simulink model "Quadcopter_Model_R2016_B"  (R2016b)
settings: Solver=VariableStepAuto  StartTime=0.0  StopTime=runtime  RelTol=1e-3
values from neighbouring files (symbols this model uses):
  delta_T = [ 0,  0,  9.404e-04 ]    [modelParameters.m]
  g = 9.81    [modelParameters.m]
  height_controlled_o = (((Rm*If        + (((omega0_o * 2 * Rm * Kv * Kq      * Kd + 1)^2) - 1)/(4* Rm*Kv^2*Kq      * Kd))/Vb)*(Pmax - Pmin) + Pmin)    [modelParameters.m]
  If = 0.3836    [modelParameters.m]
  Jreq = 4.2012e-05    [modelParameters.m]
  Jxx = 0.0110    (= 0.011)    [modelParameters.m]
  Jyy = 0.0116    [modelParameters.m]
  Jzz = 0.0223    [modelParameters.m]
  Kd = 1.4852e-07    [modelParameters.m]
  Kh = 3.4574e-04    (= 0.00034574)    [modelParameters.m]
  Kq = 96.3422    [modelParameters.m]
  Kt = 1.2007e-05    [modelParameters.m]
  Kv = 96.3422    [modelParameters.m]
  m = 1.216    [modelParameters.m]
  omega0_o = sqrt((m*g)/(4*Kt))    [modelParameters.m]
  omega1_o = sqrt((m*g)/(4*Kt))    [modelParameters.m]
  omega2_o = sqrt((m*g)/(4*Kt))    [modelParameters.m]
  omega3_o = sqrt((m*g)/(4*Kt))    [modelParameters.m]
  pitch_o = 0    [modelParameters.m]
  pitchrate_o = 0    [modelParameters.m]
  Pmax = 1    [modelParameters.m]
  Pmin = 0    [modelParameters.m]
  r_oc = [ 0 ; 0 ; 0 ]    [modelParameters.m]
  rhx = 0.16    [modelParameters.m]
  rhy = 0.16    [modelParameters.m]
  rhz = 0.03    [modelParameters.m]
  Rm = 0.235    [modelParameters.m]
  roll_o = 0    [modelParameters.m]
  rollrate_o = 0    [modelParameters.m]
  Tc = 0.01    [modelParameters.m]
  Tq = 0.005    [modelParameters.m]
  Vb = 12.3    [modelParameters.m]
  x_controlled_o = 0    [modelParameters.m]
  x_o = 0    [modelParameters.m]
  x_vel_o = 0    [modelParameters.m]
  y_controlled_o = 0    [modelParameters.m]
  y_o = 0    [modelParameters.m]
  y_vel_o = 0    [modelParameters.m]
  yaw_controlled_o = 0    [modelParameters.m]
  yaw_o = 0    [modelParameters.m]
  yawrate_o = 0    [modelParameters.m]
  z_o = 0    [modelParameters.m]
  z_vel_o = 0    [modelParameters.m]
undefined symbols (not defined in the file or in its folder): Ki, Kp, Ts
libraries: simulink x16, Derivative x13, dsparch4 x3, vrlib x1
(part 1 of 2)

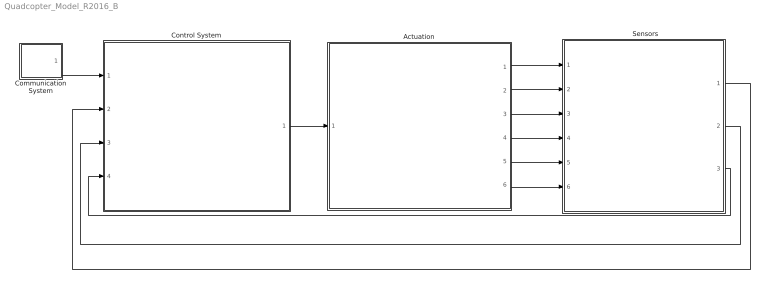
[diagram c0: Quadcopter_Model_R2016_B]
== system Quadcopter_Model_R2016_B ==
  "     Sensors   " : Subsystem
  Actuation : Subsystem
  Communication System : Subsystem
  Control System : Subsystem
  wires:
  Control System/1(P) -> Actuation/1(P)
  Actuation/6(B_g) -> "     Sensors   "/6(B_g)
  Actuation/5(B_vo_dot) -> "     Sensors   "/5(B_vo_dot)
  Actuation/4(E_ro) -> "     Sensors   "/4(E_ro)
  Actuation/3(B_vo) -> "     Sensors   "/3(B_vo)
  Actuation/1(B_omega) -> "     Sensors   "/1(B_Omega)
  "     Sensors   "/3(current_position) -> Control System/4(current_position)
  "     Sensors   "/2(euler_rates) -> Control System/3(euler_rates)
  "     Sensors   "/1(euler_angles_filtered) -> Control System/2(euler_angles_filtered)
  Actuation/2(euler_angles) -> "     Sensors   "/2(euler_angles)
  Communication System/1(setpoints) -> Control System/1(setpoints)

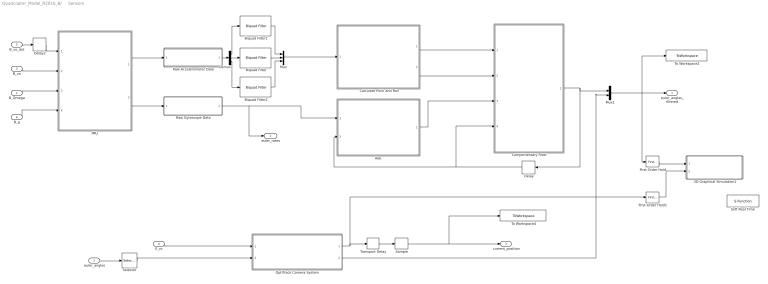
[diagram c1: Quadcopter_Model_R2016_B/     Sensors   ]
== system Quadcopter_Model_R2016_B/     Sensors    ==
  B_Omega : Inport
  euler_angles : Inport  Port=2
  B_vo : Inport  Port=3
  E_ro : Inport  Port=4
  B_vo_dot : Inport  Port=5
  B_g : Inport  Port=6
  3D Graphical Simulation1 : Subsystem
  "Aeb " : MATLAB Function  TreatAsAtomicUnit=on
  Biquad Filter : dsparch4/Biquad Filter  IIRFiltStruct=Direct form II  CoeffSource=Specify via dialog  BiQuadCoeffs=accel_SOS_Matrix  a0Flag=Warning  IC=0  ICnum=0  ICden=0  InputProcessing=Columns as channels (frame based)  denAccumFracLength=30  denProdOutputFracLength=30  secondMemoryFracLength=15  roundingMode=Floor  overflowMode=off  ScaleValues=1  optimizeScaleValues=on  ScaleValueMode=Specify via input port (g)  scaleValueFracLength=14  FilterSource=Specify via dialog  FilterObject=BQF
  Biquad Filter1 : dsparch4/Biquad Filter  IIRFiltStruct=Direct form II  CoeffSource=Specify via dialog  BiQuadCoeffs=accel_SOS_Matrix  a0Flag=Warning  IC=0  ICnum=0  ICden=0  InputProcessing=Columns as channels (frame based)  denAccumFracLength=30  denProdOutputFracLength=30  secondMemoryFracLength=15  roundingMode=Floor  overflowMode=off  ScaleValues=1  optimizeScaleValues=on  ScaleValueMode=Specify via input port (g)  scaleValueFracLength=14  FilterSource=Specify via dialog  FilterObject=BQF
  Biquad Filter2 : dsparch4/Biquad Filter  IIRFiltStruct=Direct form II  CoeffSource=Specify via dialog  BiQuadCoeffs=accel_SOS_Matrix  a0Flag=Warning  IC=0  ICnum=0  ICden=0  InputProcessing=Columns as channels (frame based)  denAccumFracLength=30  denProdOutputFracLength=30  secondMemoryFracLength=15  roundingMode=Floor  overflowMode=off  ScaleValues=1  optimizeScaleValues=on  ScaleValueMode=Specify via input port (g)  scaleValueFracLength=14  FilterSource=Specify via dialog  FilterObject=BQF
  Calculate Pitch and Roll : MATLAB Function  TreatAsAtomicUnit=on
  Complimentary Filter : MATLAB Function  TreatAsAtomicUnit=on
  Delay : Delay  DelayLength=1  InitialCondition=0
  Delay2 : Delay  DelayLength=1  InitialCondition=0  SampleTime=Tq
  Demux : Demux  Outputs=3
  First-Order Hold : simulink/Discrete/First-Order Hold  DisableCoverage=on  Ts=5e-3
  First-Order Hold1 : simulink/Discrete/First-Order Hold  DisableCoverage=on  Ts=5e-3
  "IMU " : Subsystem
  Mux : Mux  Inputs=3
  Mux1 : Mux  Inputs=2
  "OptiTrack Camera System " : Subsystem
  Raw Accelerometer Data : Subsystem  Variant=on
  Raw Gyroscope Data : Subsystem  Variant=on
  Sample : ZeroOrderHold  SampleTime=Tc
  Selector : Selector  InputPortWidth=3  IndexOptions=Index vector (dialog)  Indices=[3]  OutputSizes=1
  Soft Real Time : S-Function  Commented=on  FunctionName=sfun_time  Parameters=x  SFunctionDeploymentMode=off  EnableBusSupport=off
  To Workspace2 : ToWorkspace  VariableName=angle_IMU_reading  SaveFormat=Structure With Time  SampleTime=Tq
  To Workspace4 : ToWorkspace  VariableName=position_model  SaveFormat=Structure With Time  SampleTime=Tc
  Transport Delay : TransportDelay  DelayTime=6e-3
  euler_angles_filtered : Outport
  euler_rates : Outport  Port=2
  current_position : Outport  Port=3
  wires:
  "IMU "/1(accelerometer) -> Raw Accelerometer Data/1(raw_accel_model)
  "IMU "/2(gyroscope) -> Raw Gyroscope Data/1(raw_gyro_model)
  B_vo/1 -> "IMU "/2(B_vo)
  B_Omega/1 -> "IMU "/3(B_Omega)
  B_g/1 -> "IMU "/4(B_g)
  Calculate Pitch and Roll/2(accel_roll) -> Complimentary Filter/2(accel_roll)
  Calculate Pitch and Roll/1(accel_pitch) -> Complimentary Filter/1(accel_pitch)
  First-Order Hold/1 -> 3D Graphical Simulation1/1("Euler Angles ")
  E_ro/1 -> "OptiTrack Camera System "/1(E_ro)
  First-Order Hold1/1 -> 3D Graphical Simulation1/2(Displacement)
  B_vo_dot/1 -> Delay2/1
  Delay2/1 -> "IMU "/1(B_vo_dot)
  "OptiTrack Camera System "/1(E_ro_camera) -> Transport Delay/1, First-Order Hold1/1
  Transport Delay/1 -> Sample/1
  Sample/1 -> To Workspace4/1, current_position/1
  Raw Gyroscope Data/1(raw_gyro) -> "Aeb "/1(gyro_reading), euler_rates/1
  Delay/1 -> Complimentary Filter/4(prev_euler_angles), "Aeb "/2(euler_angles_filtered)
  "OptiTrack Camera System "/2(yaw_camera) -> Mux1/2
  "Aeb "/1(euler_rates_IMU) -> Complimentary Filter/3(euler_rates_gyro)
  Raw Accelerometer Data/1(raw_accel) -> Demux/1
  Demux/2 -> Biquad Filter/1
  Demux/1 -> Biquad Filter1/1
  Demux/3 -> Biquad Filter2/1
  Biquad Filter/1 -> Mux/2
  Biquad Filter1/1 -> Mux/1
  Biquad Filter2/1 -> Mux/3
  Mux/1 -> Calculate Pitch and Roll/1(accel_reading)
  Complimentary Filter/1(euler_angles_IMU) -> Mux1/1, Delay/1
  euler_angles/1 -> Selector/1
  Selector/1 -> "OptiTrack Camera System "/2(yaw)
  Mux1/1 -> To Workspace2/1, First-Order Hold/1, euler_angles_filtered/1

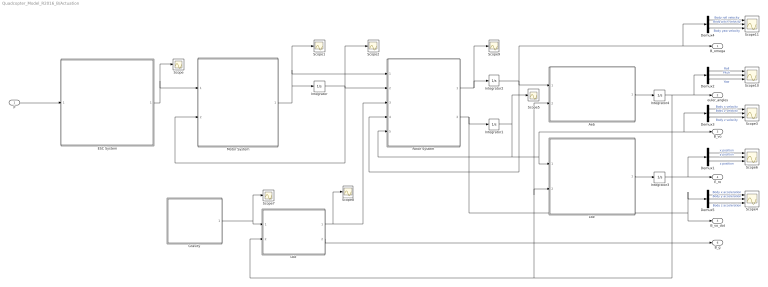
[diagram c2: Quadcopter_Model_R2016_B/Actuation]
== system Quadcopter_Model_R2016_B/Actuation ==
  P : Inport
  "Aeb " : MATLAB Function  TreatAsAtomicUnit=on
  Demux{1..5} (5 alike) : Demux  Outputs=3
  ESC System : MATLAB Function  TreatAsAtomicUnit=on
  "Gravity " : MATLAB Function  TreatAsAtomicUnit=on
  Integrator : Integrator  InitialCondition=[omega0_o, omega1_o, omega2_o, omega3_o]
  Integrator1 : Integrator  InitialCondition=[x_vel_o; y_vel_o; z_vel_o]
  Integrator2 : Integrator  InitialCondition=[rollrate_o; pitchrate_o; yawrate_o]
  Integrator3 : Integrator  InitialCondition=[x_o; y_o; z_o]
  Integrator4 : Integrator  InitialCondition=[roll_o; pitch_o; yaw_o]  ContinuousStateAttributes=['phi' 'theta' 'psi']
  "Lbe " : MATLAB Function  TreatAsAtomicUnit=on
  "Lbe " : MATLAB Function  TreatAsAtomicUnit=on
  Motor System : MATLAB Function  TreatAsAtomicUnit=on
  "Rotor System " : MATLAB Function  TreatAsAtomicUnit=on
  Scope{,1..2,5,7..9} (7 alike) : Scope
  Scope{3..4,6,10..11} (5 alike) : Scope  NumInputPorts=3
  B_omega : Outport
  euler_angles : Outport  Port=2
  B_vo : Outport  Port=3
  E_ro : Outport  Port=4
  B_vo_dot : Outport  Port=5
  B_g : Outport  Port=6
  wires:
  ESC System/1(Vb_eff) -> Scope/1, Motor System/1(Vb_eff)
  "Rotor System "/1(B_omega_dot) -> Scope9/1, Integrator2/1
  Integrator2/1 -> "Rotor System "/4(B_omega), B_omega/1, Demux4/1, "Aeb "/1(B_omega)
  "Aeb "/1(euler_rates) -> Integrator4/1
  "Lbe "/1(E_ro) -> Integrator3/1
  Integrator3/1 -> Demux1/1, E_ro/1
  "Lbe "/1(B_Fg) -> Scope8/1, "Rotor System "/3(B_Fg)
  "Lbe "/2(B_g) -> B_g/1
  Demux1/2 -> Scope6/2  "y position"
  Demux1/1 -> Scope6/1  "x position"
  Demux1/3 -> Scope6/3  "z position"
  Demux2/2 -> Scope10/2  "Pitch"
  Demux2/1 -> Scope10/1  "Roll"
  Demux2/3 -> Scope10/3  "Yaw"
  Demux4/2 -> Scope11/2  "Body pitch velocity"
  Demux4/1 -> Scope11/1  "Body roll velocity"
  Demux4/3 -> Scope11/3  "Body yaw velocity"
  Demux3/2 -> Scope3/2  "Body y velocity"
  Demux3/1 -> Scope3/1  "Body x velocity"
  Demux3/3 -> Scope3/3  "Body z velocity"
  Demux5/2 -> Scope4/2  "Body y acceleration"
  Demux5/1 -> Scope4/1  "Body x acceleration"
  Demux5/3 -> Scope4/3  "Body z acceleration"
  Integrator1/1 -> Scope5/1, "Rotor System "/5(B_vo), "Lbe "/1(B_vo), Demux3/1, B_vo/1
  "Rotor System "/2(B_vo_dot) -> Demux5/1, B_vo_dot/1, Integrator1/1
  Integrator4/1 -> euler_angles/1, Demux2/1, "Lbe "/2(euler_angles), "Aeb "/2(euler_angles), "Lbe "/2(euler_angles)
  P/1 -> ESC System/1(P)
  "Gravity "/1(E_Fg) -> Scope7/1, "Lbe "/1(E_Fg)
  Integrator/1 -> Motor System/2(w), "Rotor System "/2(w), Scope2/1
  Motor System/1(w_dot) -> Integrator/1, Scope1/1, "Rotor System "/1(w_dot)

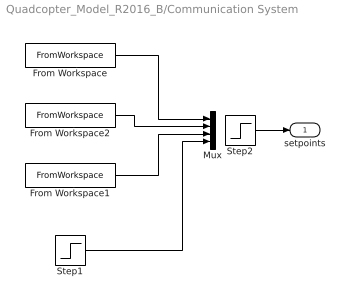
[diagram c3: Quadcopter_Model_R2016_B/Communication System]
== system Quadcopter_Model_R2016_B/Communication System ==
  From Workspace : FromWorkspace  Commented=on  VariableName=x_setpoint_model  SampleTime=Tq  Interpolate=off  OutputAfterFinalValue=Holding final value
  From Workspace1 : FromWorkspace  Commented=on  VariableName=z_setpoint_model  SampleTime=Tq  Interpolate=off  OutputAfterFinalValue=Holding final value
  From Workspace2 : FromWorkspace  Commented=on  VariableName=y_setpoint_model  SampleTime=Tq  Interpolate=off  OutputAfterFinalValue=Holding final value
  Mux : Mux
  Step1 : Step  After=0  SampleTime=0
  Step2 : Step  Before=[0,0,0,0]  After=[1,1,-1,0]  SampleTime=0
  setpoints : Outport
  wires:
  From Workspace/1 -> Mux/1
  From Workspace2/1 -> Mux/2
  From Workspace1/1 -> Mux/3
  Step1/1 -> Mux/4
  Step2/1 -> setpoints/1

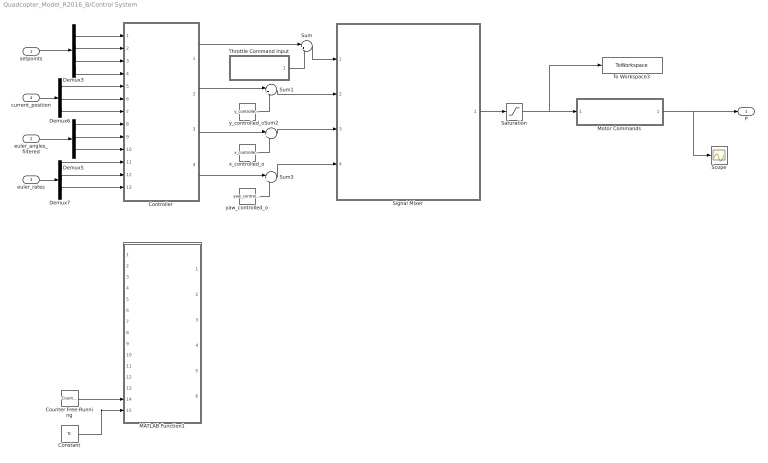
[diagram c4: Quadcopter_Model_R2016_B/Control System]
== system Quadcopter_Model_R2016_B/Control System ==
  setpoints : Inport
  euler_angles_filtered : Inport  Port=2
  euler_rates : Inport  Port=3
  current_position : Inport  Port=4
  Constant : Constant  Value=Tc  SampleTime=Tc
  Controller : Subsystem
  Counter Free-Running : simulink/Sources/Counter Free-Running  NumBits=32  tsamp=Tc
  Demux3 : Demux
  Demux5 : Demux  Outputs=3
  Demux6 : Demux  Outputs=3
  Demux7 : Demux  Outputs=3
  MATLAB Function1 : MATLAB Function  Commented=on  TreatAsAtomicUnit=on  SystemSampleTime=Tq
  Motor Commands : Subsystem  Variant=on
  Saturation : Saturate  UpperLimit=Pmax*ones(4,1)  LowerLimit=Pmin*ones(4,1)
  Scope : Scope
  Signal Mixer : MATLAB Function  TreatAsAtomicUnit=on
  Sum{,1..3} (4 alike) : Sum  Inputs=|++
  Throttle Command Input : Subsystem  Variant=on
  To Workspace3 : ToWorkspace  VariableName=motorCommands  SaveFormat=Structure With Time  SampleTime=Tq
  x_controlled_o : Constant  Value=x_controlled_o
  y_controlled_o : Constant  Value=y_controlled_o
  yaw_controlled_o : Constant  Value=yaw_controlled_o
  P : Outport
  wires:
  y_controlled_o/1 -> Sum1/2
  x_controlled_o/1 -> Sum2/2
  yaw_controlled_o/1 -> Sum3/2
  Signal Mixer/1(P) -> Saturation/1
  Counter Free-Running/1 -> MATLAB Function1/14(vrpn_id)
  Constant/1 -> MATLAB Function1/15(Tc)
  Sum1/1 -> Signal Mixer/2(y_controlled)
  Sum2/1 -> Signal Mixer/3(x_controlled)
  Sum3/1 -> Signal Mixer/4(yaw_controlled)
  Motor Commands/1(z_command) -> P/1, Scope/1
  Saturation/1 -> To Workspace3/1, Motor Commands/1(z_command_model)
  setpoints/1 -> Demux3/1
  current_position/1 -> Demux6/1
  euler_angles_filtered/1 -> Demux5/1
  euler_rates/1 -> Demux7/1
  Demux3/1 -> Controller/1(x_setpoint)
  Demux3/2 -> Controller/2(y_setpoint)
  Demux3/3 -> Controller/3(z_setpoint)
  Demux3/4 -> Controller/4(yaw_setpoint)
  Demux6/1 -> Controller/5(x_position)
  Demux6/2 -> Controller/6(y_position)
  Demux6/3 -> Controller/7(z_position)
  Demux5/1 -> Controller/8(roll)
  Demux5/2 -> Controller/9(pitch)
  Demux5/3 -> Controller/10(yaw)
  Demux7/1 -> Controller/11(roll_rate)
  Demux7/2 -> Controller/12(pitch_rate)
  Demux7/3 -> Controller/13(yaw_rate)
  Controller/1(height_controlled) -> Sum/1
  Controller/2(y_controlled) -> Sum1/1
  Controller/3(x_controlled) -> Sum2/1
  Controller/4(yaw_controlled) -> Sum3/1
  Throttle Command Input/1(z_command) -> Sum/2
  Sum/1 -> Signal Mixer/1(height_controlled)

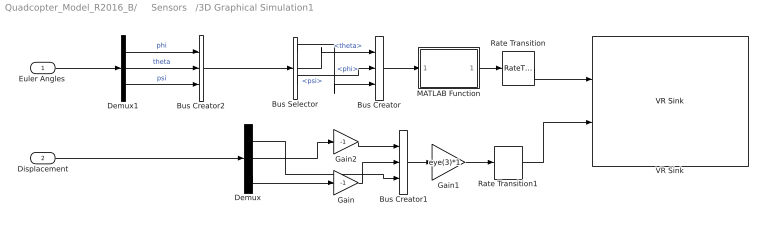
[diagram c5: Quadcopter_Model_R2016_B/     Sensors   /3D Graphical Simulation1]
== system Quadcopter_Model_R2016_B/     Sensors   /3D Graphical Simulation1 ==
  "Euler Angles " : Inport
  Displacement : Inport  Port=2
  Bus Creator : BusCreator  Inputs=3
  Bus Creator1 : BusCreator  Inputs=3
  Bus Creator2 : BusCreator  Inputs=3
  Bus Selector : BusSelector  OutputSignals=phi,theta,psi
  Demux : Demux  Outputs=3
  Demux1 : Demux  Outputs=3
  Gain : Gain  Gain=-1
  Gain1 : Gain  Gain=eye(3)*1  Multiplication=Matrix(K*u)
  Gain2 : Gain  Gain=-1
  MATLAB Function : MATLAB Function  TreatAsAtomicUnit=on
  Rate Transition : RateTransition  OutPortSampleTime=0.06
  Rate Transition1 : RateTransition  OutPortSampleTime=0.06
  VR Sink : vrlib/VR Sink  InstantiateOnLoad=on  SampleTime=-1  ViewEnable=on  RemoteChange=off  RemoteView=off  FieldsWritten=Helicopter.rotation.4.1.1.double#Helicopter.translation.3.1.1.double  WorldFileName=quadrotor_world_ucart.wrl  AutoView=on  VideoDimensions=[]  AllowVariableSize=off
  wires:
  Bus Creator2/1 -> Bus Selector/1
  Demux/1 -> Bus Creator1/3
  Gain/1 -> Bus Creator1/2
  Gain2/1 -> Bus Creator1/1
  Rate Transition1/1 -> VR Sink/2
  Rate Transition/1 -> VR Sink/1
  Demux/3 -> Gain/1
  Demux/2 -> Gain2/1
  Bus Creator1/1 -> Gain1/1
  Bus Selector/1 -> Bus Creator/3  "<phi>"
  Bus Selector/3 -> Bus Creator/2  "<psi>"
  Bus Selector/2 -> Bus Creator/1  "<theta>"
  Gain1/1 -> Rate Transition1/1
  Demux1/3 -> Bus Creator2/3  "psi"
  Demux1/2 -> Bus Creator2/2  "theta"
  Demux1/1 -> Bus Creator2/1  "phi"
  Bus Creator/1 -> MATLAB Function/1(u)
  MATLAB Function/1(y) -> Rate Transition/1
  Displacement/1 -> Demux/1
  "Euler Angles "/1 -> Demux1/1

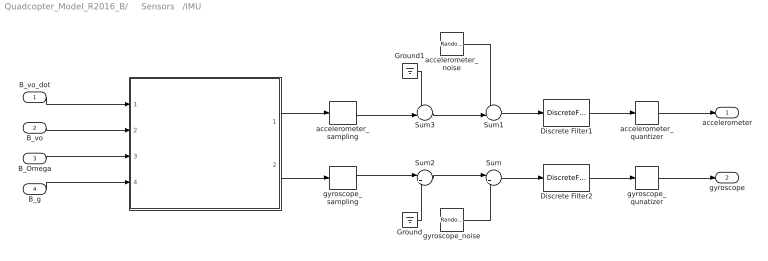
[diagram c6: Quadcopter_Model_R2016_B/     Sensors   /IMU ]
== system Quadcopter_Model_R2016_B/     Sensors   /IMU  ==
  B_vo_dot : Inport
  B_vo : Inport  Port=2
  B_Omega : Inport  Port=3
  B_g : Inport  Port=4
  " " : MATLAB Function  TreatAsAtomicUnit=on
  Discrete Filter1 : DiscreteFilter  Numerator=[0 0.749]  Denominator=[1 -0.251]  InitialStates=[0, 0, -1]  SampleTime=Tq
  Discrete Filter2 : DiscreteFilter  Numerator=[0 0.7327]  Denominator=[1 -0.2673]  SampleTime=Tq
  Ground : Ground
  Ground1 : Ground
  Sum : Sum  Inputs=|++
  Sum1 : Sum  Inputs=++|
  Sum2 : Sum  Inputs=|++
  Sum3 : Sum  Inputs=++|
  accelerometer_noise : RandomNumber  Mean=zeros(3,1)  Variance=[ 3e-7 ; 3.3e-7 ; 7.2e-7 ]  Seed=[0,1,2]  SampleTime=Tq
  accelerometer_quantizer : Quantizer  QuantizationInterval=2.4400e-04
  accelerometer_sampling : ZeroOrderHold  SampleTime=Tq
  gyroscope_noise : RandomNumber  Mean=zeros(3,1)  Variance=[ 2.2e-8 ; 1.1e-7 ; 2.4e-8 ]  Seed=[0,1,2]  SampleTime=Tq
  gyroscope_qunatizer : Quantizer  QuantizationInterval=1.1e-3
  gyroscope_sampling : ZeroOrderHold  SampleTime=Tq
  accelerometer : Outport
  gyroscope : Outport  Port=2
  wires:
  accelerometer_noise/1 -> Sum1/1
  Sum2/1 -> Sum/1
  Sum3/1 -> Sum1/2
  gyroscope_noise/1 -> Sum/2
  gyroscope_sampling/1 -> Sum2/1
  accelerometer_sampling/1 -> Sum3/2
  Ground/1 -> Sum2/2
  Ground1/1 -> Sum3/1
  B_vo_dot/1 -> " "/1(B_vo_dot)
  B_vo/1 -> " "/2(B_vo)
  B_Omega/1 -> " "/3(B_Omega)
  B_g/1 -> " "/4(B_g)
  " "/2(gyroReading) -> gyroscope_sampling/1
  " "/1(accelReading) -> accelerometer_sampling/1
  Sum1/1 -> Discrete Filter1/1
  Sum/1 -> Discrete Filter2/1
  accelerometer_quantizer/1 -> accelerometer/1
  gyroscope_qunatizer/1 -> gyroscope/1
  Discrete Filter1/1 -> accelerometer_quantizer/1
  Discrete Filter2/1 -> gyroscope_qunatizer/1

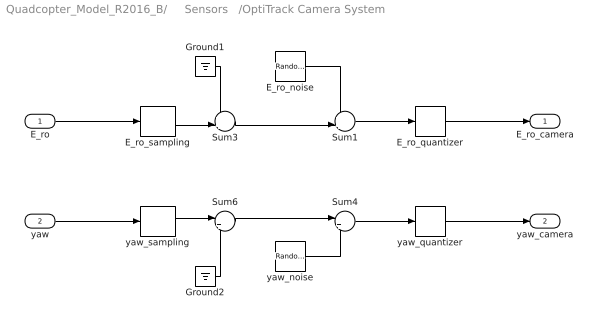
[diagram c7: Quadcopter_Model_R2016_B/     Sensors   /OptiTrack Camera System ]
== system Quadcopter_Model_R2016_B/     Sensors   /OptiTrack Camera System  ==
  E_ro : Inport
  yaw : Inport  Port=2
  E_ro_noise : RandomNumber  Mean=zeros(3,1)  Variance=[ 7.9664e-10 ; 1.1928e-10 ; 5.0636e-10 ]  Seed=[0,1,2]  SampleTime=Tc
  E_ro_quantizer : Quantizer  QuantizationInterval=2.4400e-04
  E_ro_sampling : ZeroOrderHold  SampleTime=Tc
  Ground1 : Ground
  Ground2 : Ground
  Sum1 : Sum  Inputs=++|
  Sum3 : Sum  Inputs=++|
  Sum4 : Sum  Inputs=|++
  Sum6 : Sum  Inputs=|++
  yaw_noise : RandomNumber  Variance=1.0783e-9  SampleTime=Tq
  yaw_quantizer : Quantizer  QuantizationInterval=1.1e-3
  yaw_sampling : ZeroOrderHold  SampleTime=Tq
  E_ro_camera : Outport
  yaw_camera : Outport  Port=2
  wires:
  E_ro_noise/1 -> Sum1/1
  Sum3/1 -> Sum1/2
  Sum1/1 -> E_ro_quantizer/1
  E_ro_sampling/1 -> Sum3/2
  Ground1/1 -> Sum3/1
  Sum4/1 -> yaw_quantizer/1
  Sum6/1 -> Sum4/1
  yaw_noise/1 -> Sum4/2
  yaw_sampling/1 -> Sum6/1
  Ground2/1 -> Sum6/2
  yaw/1 -> yaw_sampling/1
  E_ro/1 -> E_ro_sampling/1
  E_ro_quantizer/1 -> E_ro_camera/1
  yaw_quantizer/1 -> yaw_camera/1

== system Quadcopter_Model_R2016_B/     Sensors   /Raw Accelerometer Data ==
  note: 1) Add Subsystem or Model blocks as valid variant choices. 2) You cannot connect blocks at this level. At simulation, connectivity is automatically determined, based on the active variant and port name matching.
  raw_accel_model : Inport
  Feedback : Subsystem  VariantControl=logAnalysisToggle==0
  "Raw Accelerometer Data " : Subsystem  VariantControl=logAnalysisToggle==1
  raw_accel : Outport

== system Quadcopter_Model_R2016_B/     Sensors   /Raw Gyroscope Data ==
  note: 1) Add Subsystem or Model blocks as valid variant choices. 2) You cannot connect blocks at this level. At simulation, connectivity is automatically determined, based on the active variant and port name matching.
  raw_gyro_model : Inport
  Feedback : Subsystem  VariantControl=logAnalysisToggle==0
  "Raw Gyroscope Data " : Subsystem  VariantControl=logAnalysisToggle==1
  raw_gyro : Outport

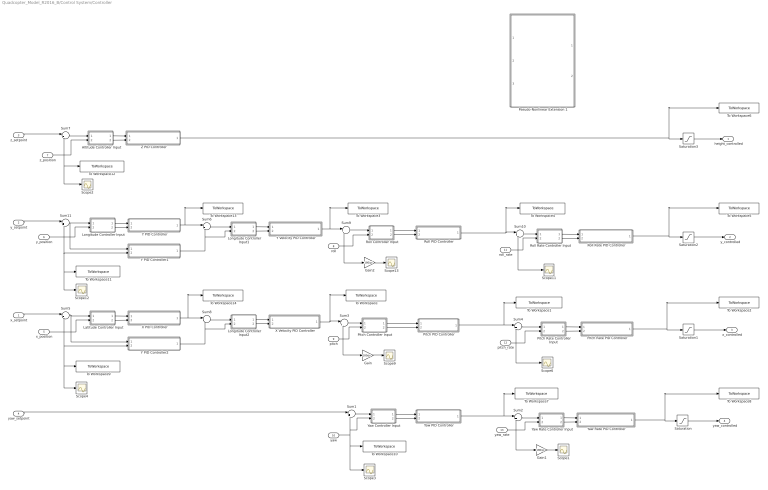
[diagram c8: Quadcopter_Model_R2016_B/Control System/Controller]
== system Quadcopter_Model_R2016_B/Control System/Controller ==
  x_setpoint : Inport
  y_setpoint : Inport  Port=2
  z_setpoint : Inport  Port=3
  yaw_setpoint : Inport  Port=4
  x_position : Inport  Port=5
  y_position : Inport  Port=6
  z_position : Inport  Port=7
  roll : Inport  Port=8
  pitch : Inport  Port=9
  yaw : Inport  Port=10
  roll_rate : Inport  Port=11
  pitch_rate : Inport  Port=12
  yaw_rate : Inport  Port=13
  Altitude Controller Input : Subsystem  Variant=on
  Gain : Gain  Gain=180/pi
  Gain1 : Gain  Gain=180/pi
  Gain2 : Gain  Gain=180/pi
  Latitude Controller Input : Subsystem  Variant=on
  Longitude Controller Input : Subsystem  Variant=on
  Longitude Controller Input1 : Subsystem  Variant=on
  Longitude Controller Input2 : Subsystem  Variant=on
  Pitch Controller Input : Subsystem  Variant=on
  Pitch PID Controller : Subsystem
  Pitch Rate Controller Input : Subsystem  Variant=on
  Pitch Rate PID Controller : Subsystem
  Pseudo-Nonlinear Extension 1 : MATLAB Function  TreatAsAtomicUnit=on
  Roll Controller Input : Subsystem  Variant=on
  Roll PID Controller : Subsystem
  Roll Rate Controller Input : Subsystem  Variant=on
  Roll Rate PID Controller : Subsystem
  Saturation{,1..3} (4 alike) : Saturate  UpperLimit=20000  LowerLimit=-20000
  Scope{1..4,6,9,11..13} (9 alike) : Scope
  Sum{1..11} (11 alike) : Sum  Inputs=|+-
  To Workspace : ToWorkspace  VariableName=pitch_setpoint_model  SaveFormat=Structure With Time  SampleTime=-1
  To Workspace1 : ToWorkspace  VariableName=pitchrate_setpoint_model  SaveFormat=Structure With Time  SampleTime=Tq
  To Workspace10 : ToWorkspace  VariableName=yaw_value_model  SaveFormat=Structure With Time  SampleTime=Tc
  To Workspace11 : ToWorkspace  VariableName=y_position_model  SaveFormat=Structure With Time  SampleTime=Tc
  To Workspace12 : ToWorkspace  VariableName=z_position_model  SaveFormat=Structure With Time  SampleTime=Tc
  To Workspace13 : ToWorkspace  VariableName=y_vel_setpoint_model  SaveFormat=Structure With Time  SampleTime=Tc
  To Workspace14 : ToWorkspace  VariableName=x_vel_setpoint_model  SaveFormat=Structure With Time  SampleTime=Tc
  To Workspace2 : ToWorkspace  VariableName=x_command_model  SaveFormat=Structure With Time  SampleTime=Tq
  To Workspace3 : ToWorkspace  VariableName=roll_setpoint_model  SaveFormat=Structure With Time  SampleTime=Tc
  To Workspace4 : ToWorkspace  VariableName=rollrate_setpoint_model  SaveFormat=Structure With Time  SampleTime=Tq
  To Workspace5 : ToWorkspace  VariableName=y_command_model  SaveFormat=Structure With Time  SampleTime=Tq
  To Workspace6 : ToWorkspace  VariableName=z_command_model  SaveFormat=Structure With Time  SampleTime=Tc
  To Workspace7 : ToWorkspace  VariableName=yawrate_setpoint_model  SaveFormat=Structure With Time  SampleTime=Tc
  To Workspace8 : ToWorkspace  VariableName=yaw_command_model  SaveFormat=Structure With Time  SampleTime=Tq
  To Workspace9 : ToWorkspace  VariableName=x_position_model  SaveFormat=Structure With Time  SampleTime=Tc
  X PID Controller : Subsystem
  X Velocity PID Controller : Subsystem
  Y PID Controller : Subsystem
  Y PID Controller1 : Subsystem
  Y PID Controller2 : Subsystem
  Y Velocity PID Controller : Subsystem
  Yaw Controller Input : Subsystem  Variant=on
  Yaw PID Controller : Subsystem
  Yaw Rate Controller Input : Subsystem  Variant=on
  Yaw Rate PID Controller : Subsystem
  Z PID Controller : Subsystem
  height_controlled : Outport
  y_controlled : Outport  Port=2
  x_controlled : Outport  Port=3
  yaw_controlled : Outport  Port=4
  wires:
  pitch_rate/1 -> Pitch Rate Controller Input/2(pitchrate_model), Scope6/1, Sum4/2
  z_setpoint/1 -> Sum7/1
  x_position/1 -> Sum5/2, Latitude Controller Input/2(x_position_model), Scope4/1, To Workspace9/1, Y PID Controller2/2(x_pos)
  Pitch PID Controller/1(pitchrate_setpoint) -> Sum4/1, To Workspace1/1
  pitch/1 -> Pitch Controller Input/2(pitch_angle_model), Gain/1, Sum3/2
  Gain/1 -> Scope9/1
  Yaw Rate PID Controller/1(yaw_motor_command) -> To Workspace8/1, Saturation/1
  Pitch Rate PID Controller/1(x_motor_command) -> Saturation1/1, To Workspace2/1
  x_setpoint/1 -> Sum5/1
  roll_rate/1 -> Roll Rate Controller Input/2(rollrate_model), Scope11/1, Sum10/2
  Roll PID Controller/1(rollrate_setpoint) -> Sum10/1, To Workspace4/1
  roll/1 -> Roll Controller Input/2(roll_angle_model), Gain2/1, Sum9/2
  Gain2/1 -> Scope13/1
  y_setpoint/1 -> Sum11/1
  yaw/1 -> Yaw Controller Input/2(yaw_angle_model), Sum1/2, Scope3/1, To Workspace10/1
  yaw_setpoint/1 -> Sum1/1
  yaw_rate/1 -> Gain1/1, Yaw Rate Controller Input/2(yawrate_model), Sum2/2
  Gain1/1 -> Scope1/1
  Yaw PID Controller/1(yawrate_setpoint) -> Sum2/1, To Workspace7/1
  z_position/1 -> Altitude Controller Input/2(z_position_model), To Workspace12/1, Scope2/1, Sum7/2
  Sum1/1 -> Yaw Controller Input/1(yaw_error_model)
  Sum2/1 -> Yaw Rate Controller Input/1(yawrate_error_model)
  Sum5/1 -> Latitude Controller Input/1(x_error_model), Y PID Controller2/1(x_error)
  Sum3/1 -> Pitch Controller Input/1(pitch_error_model)
  Sum4/1 -> Pitch Rate Controller Input/1(pitchrate_error_model)
  Sum9/1 -> Roll Controller Input/1(roll_error_model)
  Sum10/1 -> Roll Rate Controller Input/1(rollrate_error_model)
  Sum7/1 -> Altitude Controller Input/1(z_error_model)
  Roll Rate PID Controller/1(y_motor_command) -> To Workspace5/1, Saturation2/1
  Saturation3/1 -> height_controlled/1
  Saturation2/1 -> y_controlled/1
  Saturation1/1 -> x_controlled/1
  Saturation/1 -> yaw_controlled/1
  Longitude Controller Input/2(y_position) -> Y PID Controller/2(y_pos)
  Longitude Controller Input/1(y_error) -> Y PID Controller/1(y_error)
  y_position/1 -> Longitude Controller Input/2(y_position_model), Y PID Controller1/2(y_pos), To Workspace11/1, Scope12/1, Sum11/2
  Latitude Controller Input/1(x_error) -> X PID Controller/1(x_error)
  Latitude Controller Input/2(x_position) -> X PID Controller/2(x_pos)
  Yaw Controller Input/1(yaw_error) -> Yaw PID Controller/1(yaw_error)
  Yaw Controller Input/2(yaw_angle) -> Yaw PID Controller/2(yaw_angle)
  Altitude Controller Input/1(z_error) -> Z PID Controller/1(z_error)
  Altitude Controller Input/2(z_position) -> Z PID Controller/2(z_pos)
  Pitch Controller Input/1(pitch_error) -> Pitch PID Controller/1(pitch_error)
  Pitch Controller Input/2(pitch_angle) -> Pitch PID Controller/2(pitch_angle)
  Yaw Rate Controller Input/1(yawrate_error) -> Yaw Rate PID Controller/1(yawrate_error)
  Yaw Rate Controller Input/2(yawrate) -> Yaw Rate PID Controller/2(yawrate)
  Pitch Rate Controller Input/1(pitchrate_error) -> Pitch Rate PID Controller/1(pitchrate_error)
  Pitch Rate Controller Input/2(pitchrate) -> Pitch Rate PID Controller/2(pitchrate)
  Roll Controller Input/1(roll_error) -> Roll PID Controller/1(roll_error)
  Roll Controller Input/2(roll_angle) -> Roll PID Controller/2(roll_angle)
  Roll Rate Controller Input/1(rollrate_error) -> Roll Rate PID Controller/1(rollrate_error)
  Roll Rate Controller Input/2(rollrate) -> Roll Rate PID Controller/2(rollrate)
  Sum11/1 -> Longitude Controller Input/1(y_error_model), Y PID Controller1/1(y_error)
  Y PID Controller/1(roll_setpoint) -> To Workspace13/1, Sum6/1
  Y PID Controller1/1(y_vel_setpoint) -> Longitude Controller Input1/2(y_vel_model), Sum6/2
  Sum6/1 -> Longitude Controller Input1/1(y_vel_error_model)
  Longitude Controller Input1/1(y_vel_error) -> Y Velocity PID Controller/1(y_error)
  Longitude Controller Input1/2(y_vel) -> Y Velocity PID Controller/2(y_pos)
  X PID Controller/1(pitch_setpoint) -> To Workspace14/1, Sum8/1
  Y PID Controller2/1(x_vel_setpoint) -> Longitude Controller Input2/2(x_vel_model), Sum8/2
  Sum8/1 -> Longitude Controller Input2/1(x_vel_error_model)
  Longitude Controller Input2/1(x_vel_error) -> X Velocity PID Controller/1(x_vel_error)
  Longitude Controller Input2/2(x_vel) -> X Velocity PID Controller/2(x_vel)
  Z PID Controller/1(z_motor_command) -> To Workspace6/1, Saturation3/1
  Y Velocity PID Controller/1(roll_setpoint) -> To Workspace3/1, Sum9/1
  X Velocity PID Controller/1(pitch_setpoint) -> To Workspace/1, Sum3/1

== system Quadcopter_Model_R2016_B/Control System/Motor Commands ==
  note: 1) Add Subsystem or Model blocks as valid variant choices. 2) You cannot connect blocks at this level. At simulation, connectivity is automatically determined, based on the active variant and port name matching.
  z_command_model : Inport
  Feedback : Subsystem  VariantControl=logAnalysisToggle==0
  Motor Command : Subsystem  VariantControl=logAnalysisToggle==1
  z_command : Outport

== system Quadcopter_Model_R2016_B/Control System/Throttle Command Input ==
  note: 1) Add Subsystem or Model blocks as valid variant choices. 2) You cannot connect blocks at this level. At simulation, connectivity is automatically determined, based on the active variant and port name matching.
  Auto Takeoff : Subsystem  VariantControl=logAnalysisToggle==1
  height_controlled_o : Subsystem  VariantControl=logAnalysisToggle==0
  z_command : Outport

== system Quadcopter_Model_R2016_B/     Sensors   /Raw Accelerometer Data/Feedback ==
  raw_accel_model : Inport
  raw_accel : Outport
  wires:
  raw_accel_model/1 -> raw_accel/1

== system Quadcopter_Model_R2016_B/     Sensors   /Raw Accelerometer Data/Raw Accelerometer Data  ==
  From Workspace5 : FromWorkspace  VariableName=raw_accel_data  SampleTime=Tq
  raw_accel : Outport
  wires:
  From Workspace5/1 -> raw_accel/1

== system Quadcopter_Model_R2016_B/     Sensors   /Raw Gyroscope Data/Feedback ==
  raw_gyro_model : Inport
  raw_gyro : Outport
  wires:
  raw_gyro_model/1 -> raw_gyro/1

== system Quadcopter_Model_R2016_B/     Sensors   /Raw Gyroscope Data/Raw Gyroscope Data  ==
  From Workspace5 : FromWorkspace  VariableName=raw_gyro_data  SampleTime=Tq
  raw_gyro : Outport
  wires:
  From Workspace5/1 -> raw_gyro/1

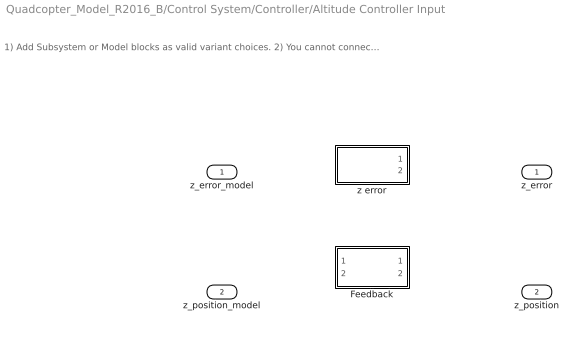
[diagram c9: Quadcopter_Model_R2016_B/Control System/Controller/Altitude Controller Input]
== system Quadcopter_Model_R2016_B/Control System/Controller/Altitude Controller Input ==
  note: 1) Add Subsystem or Model blocks as valid variant choices. 2) You cannot connect blocks at this level. At simulation, connectivity is automatically determined, based on the active variant and port name matching.
  z_error_model : Inport
  z_position_model : Inport  Port=2
  Feedback : Subsystem  VariantControl=logAnalysisToggle==0
  z error : Subsystem  VariantControl=logAnalysisToggle==1
  z_error : Outport
  z_position : Outport  Port=2

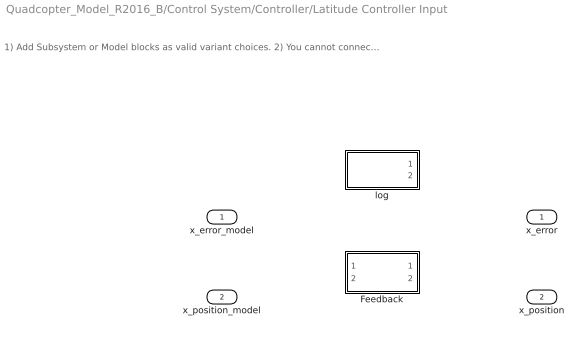
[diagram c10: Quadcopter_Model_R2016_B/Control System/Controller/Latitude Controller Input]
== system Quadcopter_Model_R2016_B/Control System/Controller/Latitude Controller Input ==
  note: 1) Add Subsystem or Model blocks as valid variant choices. 2) You cannot connect blocks at this level. At simulation, connectivity is automatically determined, based on the active variant and port name matching.
  x_error_model : Inport
  x_position_model : Inport  Port=2
  Feedback : Subsystem  VariantControl=logAnalysisToggle==0
  log : Subsystem  VariantControl=logAnalysisToggle==1
  x_error : Outport
  x_position : Outport  Port=2

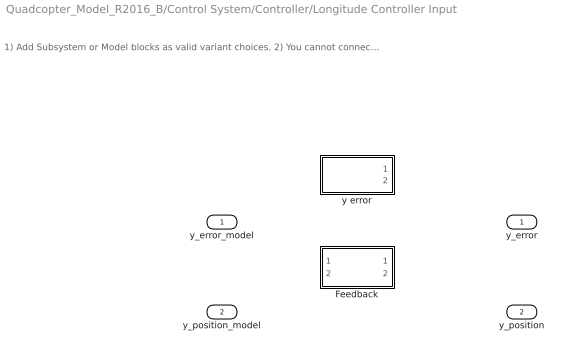
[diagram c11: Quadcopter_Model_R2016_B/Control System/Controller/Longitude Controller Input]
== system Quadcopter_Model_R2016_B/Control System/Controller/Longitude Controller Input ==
  note: 1) Add Subsystem or Model blocks as valid variant choices. 2) You cannot connect blocks at this level. At simulation, connectivity is automatically determined, based on the active variant and port name matching.
  y_error_model : Inport
  y_position_model : Inport  Port=2
  Feedback : Subsystem  VariantControl=logAnalysisToggle==0
  y error : Subsystem  VariantControl=logAnalysisToggle==1
  y_error : Outport
  y_position : Outport  Port=2

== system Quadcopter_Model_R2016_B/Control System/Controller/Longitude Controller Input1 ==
  note: 1) Add Subsystem or Model blocks as valid variant choices. 2) You cannot connect blocks at this level. At simulation, connectivity is automatically determined, based on the active variant and port name matching.
  y_vel_error_model : Inport
  y_vel_model : Inport  Port=2
  Feedback : Subsystem  VariantControl=logAnalysisToggle==0
  y error : Subsystem  VariantControl=logAnalysisToggle==1
  y_vel_error : Outport
  y_vel : Outport  Port=2

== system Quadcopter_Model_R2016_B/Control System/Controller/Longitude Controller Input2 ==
  note: 1) Add Subsystem or Model blocks as valid variant choices. 2) You cannot connect blocks at this level. At simulation, connectivity is automatically determined, based on the active variant and port name matching.
  x_vel_error_model : Inport
  x_vel_model : Inport  Port=2
  Feedback : Subsystem  VariantControl=logAnalysisToggle==0
  y error : Subsystem  VariantControl=logAnalysisToggle==1
  x_vel_error : Outport
  x_vel : Outport  Port=2

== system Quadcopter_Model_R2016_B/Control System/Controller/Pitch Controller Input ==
  note: 1) Add Subsystem or Model blocks as valid variant choices. 2) You cannot connect blocks at this level. At simulation, connectivity is automatically determined, based on the active variant and port name matching.
  pitch_error_model : Inport
  pitch_angle_model : Inport  Port=2
  Feedback : Subsystem  VariantControl=logAnalysisToggle==0
  pitch error : Subsystem  VariantControl=logAnalysisToggle==1
  pitch_error : Outport
  pitch_angle : Outport  Port=2

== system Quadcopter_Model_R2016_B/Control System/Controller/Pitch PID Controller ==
  pitch_error : Inport
  pitch_angle : Inport  Port=2
  Add : Sum  Inputs=+-
  Discrete D Controller : Derivative/Discrete D Controller  Kd=Kd  a=a
  Discrete PI Controller : simulink/Continuous/PID Controller  Controller=PI  TimeDomain=Discrete-time  SampleTime=Ts  IntegratorMethod=Forward Euler  FilterMethod=Forward Euler  Form=Parallel  UseFilter=on  ControllerParametersSource=internal  P=Kp  I=Ki  D=0  N=100  InitialConditionSource=internal  InitialConditionForIntegrator=0  InitialConditionForFilter=0  ExternalReset=none  LimitOutput=off  UpperSaturationLimit=inf  LowerSaturationLimit=-inf  LinearizeAsGain=off  AntiWindupMode=none  Kb=1  TrackingMode=off  Kt=1  PParamMin=[]  PParamMax=[]  IParamMin=[]  IParamMax=[]  DParamMin=[]  DParamMax=[]  NParamMin=[]  NParamMax=[]  KbParamMin=[]  KbParamMax=[]  KtParamMin=[]  KtParamMax=[]  POutMin=[]  POutMax=[]  IOutMin=[]  IOutMax=[]  DOutMin=[]  DOutMax=[]  NOutMin=[]  NOutMax=[]  KbOutMin=[]  KbOutMax=[]  KtOutMin=[]  KtOutMax=[]  IntegratorOutMin=[]  IntegratorOutMax=[]  FilterOutMin=[]  FilterOutMax=[]  SumOutMin=[]  SumOutMax=[]  SumI1OutMin=[]  SumI1OutMax=[]  SumI2OutMin=[]  SumI2OutMax=[]  SumI3OutMin=[]  SumI3OutMax=[]  SumDOutMin=[]  SumDOutMax=[]  SaturationOutMin=[]  SaturationOutMax=[]  IntegratorContinuousStateAttributes=''  IntegratorStateMustResolveToSignalObject=off  IntegratorRTWStateStorageClass=Auto  FilterContinuousStateAttributes=''  FilterStateMustResolveToSignalObject=off  FilterRTWStateStorageClass=Auto  DifferentiatorICPrevScaledInput=0  DifferentiatorOutMin=[]  DifferentiatorOutMax=[]
  pitchrate_setpoint : Outport
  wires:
  pitch_angle/1 -> Discrete D Controller/1
  pitch_error/1 -> Discrete PI Controller/1
  Discrete PI Controller/1 -> Add/1
  Discrete D Controller/1 -> Add/2
  Add/1 -> pitchrate_setpoint/1

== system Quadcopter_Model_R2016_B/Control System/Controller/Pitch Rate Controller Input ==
  note: 1) Add Subsystem or Model blocks as valid variant choices. 2) You cannot connect blocks at this level. At simulation, connectivity is automatically determined, based on the active variant and port name matching.
  pitchrate_error_model : Inport
  pitchrate_model : Inport  Port=2
  Feedback : Subsystem  VariantControl=logAnalysisToggle==0
  pitchrate error : Subsystem  VariantControl=logAnalysisToggle==1
  pitchrate_error : Outport
  pitchrate : Outport  Port=2

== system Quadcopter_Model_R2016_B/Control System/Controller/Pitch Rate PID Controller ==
  pitchrate_error : Inport
  pitchrate : Inport  Port=2
  Add : Sum  Inputs=+-
  Discrete D Controller : Derivative/Discrete D Controller  Kd=Kd  a=a
  Discrete PI Controller : simulink/Continuous/PID Controller  Controller=PI  TimeDomain=Discrete-time  SampleTime=Ts  IntegratorMethod=Forward Euler  FilterMethod=Forward Euler  Form=Parallel  UseFilter=on  ControllerParametersSource=internal  P=Kp  I=Ki  D=0  N=100  InitialConditionSource=internal  InitialConditionForIntegrator=0  InitialConditionForFilter=0  ExternalReset=none  LimitOutput=off  UpperSaturationLimit=inf  LowerSaturationLimit=-inf  LinearizeAsGain=off  AntiWindupMode=none  Kb=1  TrackingMode=off  Kt=1  PParamMin=[]  PParamMax=[]  IParamMin=[]  IParamMax=[]  DParamMin=[]  DParamMax=[]  NParamMin=[]  NParamMax=[]  KbParamMin=[]  KbParamMax=[]  KtParamMin=[]  KtParamMax=[]  POutMin=[]  POutMax=[]  IOutMin=[]  IOutMax=[]  DOutMin=[]  DOutMax=[]  NOutMin=[]  NOutMax=[]  KbOutMin=[]  KbOutMax=[]  KtOutMin=[]  KtOutMax=[]  IntegratorOutMin=[]  IntegratorOutMax=[]  FilterOutMin=[]  FilterOutMax=[]  SumOutMin=[]  SumOutMax=[]  SumI1OutMin=[]  SumI1OutMax=[]  SumI2OutMin=[]  SumI2OutMax=[]  SumI3OutMin=[]  SumI3OutMax=[]  SumDOutMin=[]  SumDOutMax=[]  SaturationOutMin=[]  SaturationOutMax=[]  IntegratorContinuousStateAttributes=''  IntegratorStateMustResolveToSignalObject=off  IntegratorRTWStateStorageClass=Auto  FilterContinuousStateAttributes=''  FilterStateMustResolveToSignalObject=off  FilterRTWStateStorageClass=Auto  DifferentiatorICPrevScaledInput=0  DifferentiatorOutMin=[]  DifferentiatorOutMax=[]
  x_motor_command : Outport
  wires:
  pitchrate/1 -> Discrete D Controller/1
  pitchrate_error/1 -> Discrete PI Controller/1
  Discrete PI Controller/1 -> Add/1
  Discrete D Controller/1 -> Add/2
  Add/1 -> x_motor_command/1

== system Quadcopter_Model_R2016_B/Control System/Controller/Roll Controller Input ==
  note: 1) Add Subsystem or Model blocks as valid variant choices. 2) You cannot connect blocks at this level. At simulation, connectivity is automatically determined, based on the active variant and port name matching.
  roll_error_model : Inport
  roll_angle_model : Inport  Port=2
  Feedback : Subsystem  VariantControl=logAnalysisToggle==0
  roll error : Subsystem  VariantControl=logAnalysisToggle==1
  roll_error : Outport
  roll_angle : Outport  Port=2

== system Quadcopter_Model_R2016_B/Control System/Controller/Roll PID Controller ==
  roll_error : Inport
  roll_angle : Inport  Port=2
  Add : Sum  Inputs=+-
  Discrete D Controller : Derivative/Discrete D Controller  Kd=Kd  a=a
  Discrete PI Controller : simulink/Continuous/PID Controller  Controller=PI  TimeDomain=Discrete-time  SampleTime=Ts  IntegratorMethod=Forward Euler  FilterMethod=Forward Euler  Form=Parallel  UseFilter=on  ControllerParametersSource=internal  P=Kp  I=Ki  D=0  N=100  InitialConditionSource=internal  InitialConditionForIntegrator=0  InitialConditionForFilter=0  ExternalReset=none  LimitOutput=off  UpperSaturationLimit=inf  LowerSaturationLimit=-inf  LinearizeAsGain=off  AntiWindupMode=none  Kb=1  TrackingMode=off  Kt=1  PParamMin=[]  PParamMax=[]  IParamMin=[]  IParamMax=[]  DParamMin=[]  DParamMax=[]  NParamMin=[]  NParamMax=[]  KbParamMin=[]  KbParamMax=[]  KtParamMin=[]  KtParamMax=[]  POutMin=[]  POutMax=[]  IOutMin=[]  IOutMax=[]  DOutMin=[]  DOutMax=[]  NOutMin=[]  NOutMax=[]  KbOutMin=[]  KbOutMax=[]  KtOutMin=[]  KtOutMax=[]  IntegratorOutMin=[]  IntegratorOutMax=[]  FilterOutMin=[]  FilterOutMax=[]  SumOutMin=[]  SumOutMax=[]  SumI1OutMin=[]  SumI1OutMax=[]  SumI2OutMin=[]  SumI2OutMax=[]  SumI3OutMin=[]  SumI3OutMax=[]  SumDOutMin=[]  SumDOutMax=[]  SaturationOutMin=[]  SaturationOutMax=[]  IntegratorContinuousStateAttributes=''  IntegratorStateMustResolveToSignalObject=off  IntegratorRTWStateStorageClass=Auto  FilterContinuousStateAttributes=''  FilterStateMustResolveToSignalObject=off  FilterRTWStateStorageClass=Auto  DifferentiatorICPrevScaledInput=0  DifferentiatorOutMin=[]  DifferentiatorOutMax=[]
  rollrate_setpoint : Outport
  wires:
  roll_angle/1 -> Discrete D Controller/1
  roll_error/1 -> Discrete PI Controller/1
  Discrete PI Controller/1 -> Add/1
  Discrete D Controller/1 -> Add/2
  Add/1 -> rollrate_setpoint/1

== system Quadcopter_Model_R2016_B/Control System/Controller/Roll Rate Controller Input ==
  note: 1) Add Subsystem or Model blocks as valid variant choices. 2) You cannot connect blocks at this level. At simulation, connectivity is automatically determined, based on the active variant and port name matching.
  rollrate_error_model : Inport
  rollrate_model : Inport  Port=2
  Feedback : Subsystem  VariantControl=logAnalysisToggle==0
  rollrate error : Subsystem  VariantControl=logAnalysisToggle==1
  rollrate_error : Outport
  rollrate : Outport  Port=2

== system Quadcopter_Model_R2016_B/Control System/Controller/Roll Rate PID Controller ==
  rollrate_error : Inport
  rollrate : Inport  Port=2
  Add : Sum  Inputs=+-
  Discrete D Controller : Derivative/Discrete D Controller  Kd=Kd  a=a
  Discrete PI Controller : simulink/Continuous/PID Controller  Controller=PI  TimeDomain=Discrete-time  SampleTime=Ts  IntegratorMethod=Forward Euler  FilterMethod=Forward Euler  Form=Parallel  UseFilter=on  ControllerParametersSource=internal  P=Kp  I=Ki  D=0  N=100  InitialConditionSource=internal  InitialConditionForIntegrator=0  InitialConditionForFilter=0  ExternalReset=none  LimitOutput=off  UpperSaturationLimit=inf  LowerSaturationLimit=-inf  LinearizeAsGain=off  AntiWindupMode=none  Kb=1  TrackingMode=off  Kt=1  PParamMin=[]  PParamMax=[]  IParamMin=[]  IParamMax=[]  DParamMin=[]  DParamMax=[]  NParamMin=[]  NParamMax=[]  KbParamMin=[]  KbParamMax=[]  KtParamMin=[]  KtParamMax=[]  POutMin=[]  POutMax=[]  IOutMin=[]  IOutMax=[]  DOutMin=[]  DOutMax=[]  NOutMin=[]  NOutMax=[]  KbOutMin=[]  KbOutMax=[]  KtOutMin=[]  KtOutMax=[]  IntegratorOutMin=[]  IntegratorOutMax=[]  FilterOutMin=[]  FilterOutMax=[]  SumOutMin=[]  SumOutMax=[]  SumI1OutMin=[]  SumI1OutMax=[]  SumI2OutMin=[]  SumI2OutMax=[]  SumI3OutMin=[]  SumI3OutMax=[]  SumDOutMin=[]  SumDOutMax=[]  SaturationOutMin=[]  SaturationOutMax=[]  IntegratorContinuousStateAttributes=''  IntegratorStateMustResolveToSignalObject=off  IntegratorRTWStateStorageClass=Auto  FilterContinuousStateAttributes=''  FilterStateMustResolveToSignalObject=off  FilterRTWStateStorageClass=Auto  DifferentiatorICPrevScaledInput=0  DifferentiatorOutMin=[]  DifferentiatorOutMax=[]
  y_motor_command : Outport
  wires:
  rollrate/1 -> Discrete D Controller/1
  rollrate_error/1 -> Discrete PI Controller/1
  Discrete PI Controller/1 -> Add/1
  Discrete D Controller/1 -> Add/2
  Add/1 -> y_motor_command/1

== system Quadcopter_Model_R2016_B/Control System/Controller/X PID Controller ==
  x_error : Inport
  x_pos : Inport  Port=2
  Add : Sum  Inputs=+-
  Discrete D Controller : Derivative/Discrete D Controller  Kd=Kd  a=a
  Discrete PI Controller : simulink/Continuous/PID Controller  Controller=PI  TimeDomain=Discrete-time  SampleTime=Ts  IntegratorMethod=Forward Euler  FilterMethod=Forward Euler  Form=Parallel  UseFilter=on  ControllerParametersSource=internal  P=Kp  I=Ki  D=0  N=100  InitialConditionSource=internal  InitialConditionForIntegrator=0  InitialConditionForFilter=0  ExternalReset=none  LimitOutput=off  UpperSaturationLimit=inf  LowerSaturationLimit=-inf  LinearizeAsGain=off  AntiWindupMode=none  Kb=1  TrackingMode=off  Kt=1  PParamMin=[]  PParamMax=[]  IParamMin=[]  IParamMax=[]  DParamMin=[]  DParamMax=[]  NParamMin=[]  NParamMax=[]  KbParamMin=[]  KbParamMax=[]  KtParamMin=[]  KtParamMax=[]  POutMin=[]  POutMax=[]  IOutMin=[]  IOutMax=[]  DOutMin=[]  DOutMax=[]  NOutMin=[]  NOutMax=[]  KbOutMin=[]  KbOutMax=[]  KtOutMin=[]  KtOutMax=[]  IntegratorOutMin=[]  IntegratorOutMax=[]  FilterOutMin=[]  FilterOutMax=[]  SumOutMin=[]  SumOutMax=[]  SumI1OutMin=[]  SumI1OutMax=[]  SumI2OutMin=[]  SumI2OutMax=[]  SumI3OutMin=[]  SumI3OutMax=[]  SumDOutMin=[]  SumDOutMax=[]  SaturationOutMin=[]  SaturationOutMax=[]  IntegratorContinuousStateAttributes=''  IntegratorStateMustResolveToSignalObject=off  IntegratorRTWStateStorageClass=Auto  FilterContinuousStateAttributes=''  FilterStateMustResolveToSignalObject=off  FilterRTWStateStorageClass=Auto  DifferentiatorICPrevScaledInput=0  DifferentiatorOutMin=[]  DifferentiatorOutMax=[]
  pitch_setpoint : Outport
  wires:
  x_pos/1 -> Discrete D Controller/1
  x_error/1 -> Discrete PI Controller/1
  Discrete PI Controller/1 -> Add/1
  Discrete D Controller/1 -> Add/2
  Add/1 -> pitch_setpoint/1

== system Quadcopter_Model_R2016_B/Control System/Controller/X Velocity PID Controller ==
  x_vel_error : Inport
  x_vel : Inport  Port=2
  Add : Sum  Inputs=+-
  Discrete D Controller : Derivative/Discrete D Controller  Kd=Kd  a=a
  Discrete PI Controller : simulink/Continuous/PID Controller  Controller=PI  TimeDomain=Discrete-time  SampleTime=Ts  IntegratorMethod=Forward Euler  FilterMethod=Forward Euler  Form=Parallel  UseFilter=on  ControllerParametersSource=internal  P=Kp  I=Ki  D=0  N=100  InitialConditionSource=internal  InitialConditionForIntegrator=0  InitialConditionForFilter=0  ExternalReset=none  LimitOutput=off  UpperSaturationLimit=inf  LowerSaturationLimit=-inf  LinearizeAsGain=off  AntiWindupMode=none  Kb=1  TrackingMode=off  Kt=1  PParamMin=[]  PParamMax=[]  IParamMin=[]  IParamMax=[]  DParamMin=[]  DParamMax=[]  NParamMin=[]  NParamMax=[]  KbParamMin=[]  KbParamMax=[]  KtParamMin=[]  KtParamMax=[]  POutMin=[]  POutMax=[]  IOutMin=[]  IOutMax=[]  DOutMin=[]  DOutMax=[]  NOutMin=[]  NOutMax=[]  KbOutMin=[]  KbOutMax=[]  KtOutMin=[]  KtOutMax=[]  IntegratorOutMin=[]  IntegratorOutMax=[]  FilterOutMin=[]  FilterOutMax=[]  SumOutMin=[]  SumOutMax=[]  SumI1OutMin=[]  SumI1OutMax=[]  SumI2OutMin=[]  SumI2OutMax=[]  SumI3OutMin=[]  SumI3OutMax=[]  SumDOutMin=[]  SumDOutMax=[]  SaturationOutMin=[]  SaturationOutMax=[]  IntegratorContinuousStateAttributes=''  IntegratorStateMustResolveToSignalObject=off  IntegratorRTWStateStorageClass=Auto  FilterContinuousStateAttributes=''  FilterStateMustResolveToSignalObject=off  FilterRTWStateStorageClass=Auto  DifferentiatorICPrevScaledInput=0  DifferentiatorOutMin=[]  DifferentiatorOutMax=[]
  pitch_setpoint : Outport
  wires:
  x_vel/1 -> Discrete D Controller/1
  x_vel_error/1 -> Discrete PI Controller/1
  Discrete PI Controller/1 -> Add/1
  Discrete D Controller/1 -> Add/2
  Add/1 -> pitch_setpoint/1

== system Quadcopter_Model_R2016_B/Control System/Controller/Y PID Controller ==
  y_error : Inport
  y_pos : Inport  Port=2
  Add : Sum  Inputs=+-
  Discrete D Controller : Derivative/Discrete D Controller  Kd=Kd  a=a
  Discrete PI Controller : simulink/Continuous/PID Controller  Controller=PI  TimeDomain=Discrete-time  SampleTime=Ts  IntegratorMethod=Forward Euler  FilterMethod=Forward Euler  Form=Parallel  UseFilter=on  ControllerParametersSource=internal  P=Kp  I=Ki  D=0  N=100  InitialConditionSource=internal  InitialConditionForIntegrator=0  InitialConditionForFilter=0  ExternalReset=none  LimitOutput=off  UpperSaturationLimit=inf  LowerSaturationLimit=-inf  LinearizeAsGain=off  AntiWindupMode=none  Kb=1  TrackingMode=off  Kt=1  PParamMin=[]  PParamMax=[]  IParamMin=[]  IParamMax=[]  DParamMin=[]  DParamMax=[]  NParamMin=[]  NParamMax=[]  KbParamMin=[]  KbParamMax=[]  KtParamMin=[]  KtParamMax=[]  POutMin=[]  POutMax=[]  IOutMin=[]  IOutMax=[]  DOutMin=[]  DOutMax=[]  NOutMin=[]  NOutMax=[]  KbOutMin=[]  KbOutMax=[]  KtOutMin=[]  KtOutMax=[]  IntegratorOutMin=[]  IntegratorOutMax=[]  FilterOutMin=[]  FilterOutMax=[]  SumOutMin=[]  SumOutMax=[]  SumI1OutMin=[]  SumI1OutMax=[]  SumI2OutMin=[]  SumI2OutMax=[]  SumI3OutMin=[]  SumI3OutMax=[]  SumDOutMin=[]  SumDOutMax=[]  SaturationOutMin=[]  SaturationOutMax=[]  IntegratorContinuousStateAttributes=''  IntegratorStateMustResolveToSignalObject=off  IntegratorRTWStateStorageClass=Auto  FilterContinuousStateAttributes=''  FilterStateMustResolveToSignalObject=off  FilterRTWStateStorageClass=Auto  DifferentiatorICPrevScaledInput=0  DifferentiatorOutMin=[]  DifferentiatorOutMax=[]
  roll_setpoint : Outport
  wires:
  y_pos/1 -> Discrete D Controller/1
  y_error/1 -> Discrete PI Controller/1
  Discrete PI Controller/1 -> Add/1
  Discrete D Controller/1 -> Add/2
  Add/1 -> roll_setpoint/1

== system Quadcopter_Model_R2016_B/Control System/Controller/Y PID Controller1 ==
  y_error : Inport
  y_pos : Inport  Port=2
  Add : Sum  Inputs=+-
  Discrete D Controller : Derivative/Discrete D Controller  Kd=Kd  a=a
  Discrete PI Controller : simulink/Continuous/PID Controller  Controller=PI  TimeDomain=Discrete-time  SampleTime=Ts  IntegratorMethod=Forward Euler  FilterMethod=Forward Euler  Form=Parallel  UseFilter=on  ControllerParametersSource=internal  P=Kp  I=Ki  D=0  N=100  InitialConditionSource=internal  InitialConditionForIntegrator=0  InitialConditionForFilter=0  ExternalReset=none  LimitOutput=off  UpperSaturationLimit=inf  LowerSaturationLimit=-inf  LinearizeAsGain=off  AntiWindupMode=none  Kb=1  TrackingMode=off  Kt=1  PParamMin=[]  PParamMax=[]  IParamMin=[]  IParamMax=[]  DParamMin=[]  DParamMax=[]  NParamMin=[]  NParamMax=[]  KbParamMin=[]  KbParamMax=[]  KtParamMin=[]  KtParamMax=[]  POutMin=[]  POutMax=[]  IOutMin=[]  IOutMax=[]  DOutMin=[]  DOutMax=[]  NOutMin=[]  NOutMax=[]  KbOutMin=[]  KbOutMax=[]  KtOutMin=[]  KtOutMax=[]  IntegratorOutMin=[]  IntegratorOutMax=[]  FilterOutMin=[]  FilterOutMax=[]  SumOutMin=[]  SumOutMax=[]  SumI1OutMin=[]  SumI1OutMax=[]  SumI2OutMin=[]  SumI2OutMax=[]  SumI3OutMin=[]  SumI3OutMax=[]  SumDOutMin=[]  SumDOutMax=[]  SaturationOutMin=[]  SaturationOutMax=[]  IntegratorContinuousStateAttributes=''  IntegratorStateMustResolveToSignalObject=off  IntegratorRTWStateStorageClass=Auto  FilterContinuousStateAttributes=''  FilterStateMustResolveToSignalObject=off  FilterRTWStateStorageClass=Auto  DifferentiatorICPrevScaledInput=0  DifferentiatorOutMin=[]  DifferentiatorOutMax=[]
  y_vel_setpoint : Outport
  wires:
  y_pos/1 -> Discrete D Controller/1
  y_error/1 -> Discrete PI Controller/1
  Discrete PI Controller/1 -> Add/1
  Discrete D Controller/1 -> Add/2
  Add/1 -> y_vel_setpoint/1
